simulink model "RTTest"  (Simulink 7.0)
settings: Solver=FixedStepDiscrete  StartTime=0.0  StopTime=inf  RelTol=1e-3
PreLoadFcn:
  | scramInitialize;
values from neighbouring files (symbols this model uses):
  nActSts = nAct    (= 5)    [scramInitialize.m]
  nAdcUSts = nAdcU    (= 18)    [scramInitialize.m]
  nDoutSts = nDout    (= 4)    [scramInitialize.m]
  nEncUSts = nEncU    (= 4)    [scramInitialize.m]
  nodeMats = node    [scramInitialize.m]
  nodeSts = node    [scramInitialize.m]
  nTblMats = nTbl    (= 6)    [scramInitialize.m]
  samplePeriod = 1/1024    (= 0.0009765625)    [scramInitialize.m]    (also in viewer.m = eval(getHeaderValue(header, 'DELTA_T')))
undefined symbols (not defined in the file or in its folder): DiscIntNeverNeededParam, Flat
libraries: xpcsystranlib x5, xpclib x5, simulink x1

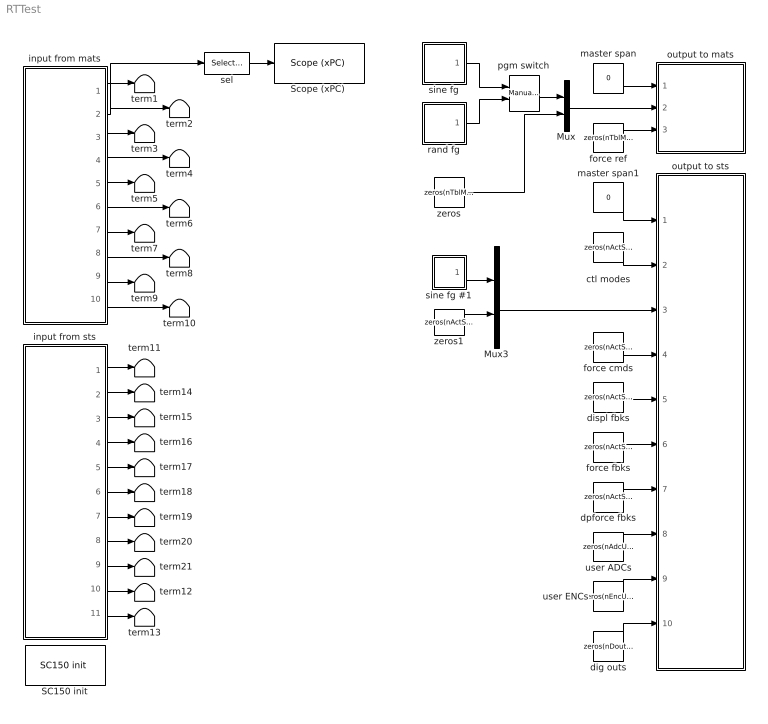
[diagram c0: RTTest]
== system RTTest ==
  Mux : Mux  Inputs=2
  Mux3 : Mux  Inputs=2
  SC150 init : xpcsystranlib/Shared Memory/SC150 init   node=node  pci=-1
  "Scope (xPC) " : xpclib/Misc./Scope (xPC)   SystemSampleTime=-1  scopeno=1  scopetype=Target  autostart=on  viewmode=Graphical redraw  formatstr='%15.6f'  grid=on  ylimits=[0,0]  nosamples=1024  noprepostsamples=0  interleave=1  triggermode=FreeRun  triggersignal=1  triggerlevel=0.0  triggerslope=Either  triggerscope=1  triggersample=0  filename=data.dat  mode=Lazy  writesize=512  autorestart=off
  ctl modes : Constant  Value=zeros(nActSts, 1)  OutDataType=sfix(16)  OutScaling=2^0
  dig outs : Constant  Value=zeros(nDoutSts, 1)  OutDataTypeMode=uint32  OutDataType=sfix(16)  OutScaling=2^0
  displ fbks : Constant  Value=zeros(nActSts, 1)  OutDataType=sfix(16)  OutScaling=2^0
  dpforce fbks : Constant  Value=zeros(nActSts, 1)  OutDataType=sfix(16)  OutScaling=2^0
  force cmds : Constant  Value=zeros(nActSts, 1)  OutDataType=sfix(16)  OutScaling=2^0
  force fbks : Constant  Value=zeros(nActSts, 1)  OutDataType=sfix(16)  OutScaling=2^0
  force ref : Constant  Value=zeros(nTblMats, 1)  OutDataType=sfix(16)  OutScaling=2^0
  input from mats : Subsystem
  input from sts : Subsystem
  master span : Constant  Value=0  OutDataType=sfix(16)  OutScaling=2^0
  master span1 : Constant  Value=0  OutDataType=sfix(16)  OutScaling=2^0
  output to mats : Subsystem
  output to sts : Subsystem
  pgm switch : simulink/Signal Routing/Manual Switch  SystemSampleTime=-1  sw=1  action=0  varsize=off
  rand fg : Subsystem  mask(Random Function Generator){shape=Flat, ampl=0.05, minFreq=0, maxFreq=10, spanInterval=1, samplePeriod=samplePeriod, showFRF=off}
      mask prompts: ampl "RMS amplitude"; minFreq "Minimum frequency (Hz)"; maxFreq "Maximum frequency (Hz)"; spanInterval "Span interval (sec)"; samplePeriod "Sample period (sec)"; showFRF "Show filter frequency response"
      mask init:
      | fsamp	= 1 / samplePeriod;
      | 
      | % design shaping filter
      | switch (shape)
      | 	case '1/F^2'	% 1/f^2 (two-pole lowpass)
      | 		% Note: Has unity amplitude at minFreq, then
      | 		% decreases at -40db per decade up to maxFreq.
      | 		minFreq = max(minFreq, 0.01*maxFreq);
      | 		k		= 0.1;
      | 		fpass	= k * minFreq;
      | 		alpha	= -exp(-2 * pi * fpass / fsamp);
      | 		a1		= 2 * alpha;
      | 		a2		= alpha^2;
      | 		b0		= (1/k)^2 * (1 + a1 + a2) * 0.25;
      | 		b1		= 2 * b0
      | 		b2		= b0
      | 		noiseBw = (minFreq / 3) * (1 - (minFreq / maxFreq)^3);
      | 	case '1/F'		% 1/f (one-pole lowpass)
      | 		% Note: Has unity amplitude at minFreq, then
      | 		% decreases at -20db per decade up to maxFreq.
      | 		minFreq = max(minFreq, 0.01*maxFreq);
      | 		k		= 0.1;
      | 		fpass	= k * minFreq;
      | 		alpha	= -exp(-2 * pi * fpass / fsamp);
      | 		a1		= alpha;
      | 		a2		= 0;
      | 		b0		= (1/k) * (1 + a1) * 0.5;
      | 		b1		= b0;
      | 		b2		= 0;
      | 		noiseBw = minFreq * (1 - (minFreq / maxFreq));
      | 	case 'Flat'		% flat
      | 		fpass	= maxFreq;
      | 		a1		= 0;
      | 		a2		= 0;
      | 		b0		= 1;
      | 		b1		= 0;
      | 		b2		= 0;
      | 		noiseBw = maxFreq - minFreq;
      | 	case 'F'		% f (single differentiator)
      | 		% Note:  A simple backward difference is a valid
      | 		% differentiator only up to about one half of nyquist.
      | 		% So we will select coefficients so that the slope,
      | 		% if extrapolated, would reach unity gain at nyquist
      | 		% (in reality, the gain will fall short of unity).
      | 		% These coefficients will be experimentally determined.
      | 		a1		= 0;
      | 		a2		= 0;
      | 		b0		= 0.33;
      | 		b1		= -b0;
      | 		b2		= 0;
      | 		noiseBw	= (4/3) * (maxFreq*(maxFreq/fsamp)^2 - minFreq*(minFreq/fsamp)^2);
      | 	case 'F^2'		% f^2 (double differentiator)
      | 		% Note:  See note above.
      | 		a1		= 0;
      | 		a2		= 0;
      | 		b0		= (0.33)^2;
      | 		b1		= -2 * b0;
      | 		b2		= b0;
      | 		noiseBw = (16/5) * (maxFreq*(maxFreq/fsamp)^4 - minFreq*(minFreq/fsamp)^4);
      | end
      | aSpf = [1 a1 a2];
      | bSpf = [b0 b1 b2];
      | peakAmpl = ampl * sqrt(3) * sqrt(max(0.5*fsamp/noiseBw, 1));
      | 
      | % design bandlimiting filter
      | fpassU	= maxFreq;
      | fstopU	= fpassU * 1.25;
      | fpassL	= min(minFreq, fpassU-0.001);
      | fstopL	= fpassL * 0.5;
      | rpass	= 0.01;
      | rstop	= 0.01;
      | rpassDB	= -20*log10(1-rpass);
      | rstopDB	= -20*log10(rstop);
      | bHpf	= [1];
      | aHpf	= [1];
      | bLpf	= [1];
      | aLpf	= [1];
      | if fpassL == 0
      | 		if fstopU < 0.5 * fsamp		% lowpass
      | 			[n, wn]	= ellipord(2*fpassU/fsamp, 2*fstopU/fsamp, rpassDB, rstopDB);
      | 			[bLpf, aLpf] = ellip(n, rpassDB, rstopDB, wn, 'low');
      | 		end
      | else
      | 		if fstopU < 0.5 * fsamp		% bandpass (implemented as series HP & LP)
      | 			rpassDB = rpassDB / 2;
      | 			[n, wn]	= ellipord(2*fpassU/fsamp, 2*fstopU/fsamp, rpassDB, rstopDB);
      | 			[bLpf, aLpf] = ellip(n, rpassDB, rstopDB, wn, 'low');
      | 			[n, wn]	= ellipord(2*fpassL/fsamp, 2*fstopL/fsamp, rpassDB, rstopDB);
      | 			[bHpf, aHpf] = ellip(n, rpassDB, rstopDB, wn, 'high');
      | 		else						% highpass
      | 			[n, wn]	= ellipord(2*fpassU/fsamp, 2*fstopU/fsamp, rpassDB, rstopDB);
      | 			[bHpf, aHpf] = ellip(n, rpassDB, rstopDB, wn, 'high');
      | 		end	
      | end
      | if showFRF
      | 	f     = linspace(0, fsamp/4, 8192);
      | 	tfSpf = freqz(bSpf, aSpf, f, fsamp);
      | 	tfLpf = freqz(bLpf, aLpf, f, fsamp);
      | 	tfHpf = freqz(bHpf, aHpf, f, fsamp);
      | 	plot(f, 20*log10(peakAmpl*abs(tfSpf.*tfLpf.*tfHpf)));
      | 	title('Filter Frequency Response');
      | 	ylabel('dB');
      | 	xlabel('Hz');
      | end
  sel : Selector  IndexOptions=Index vector (dialog)  Indices=1  OutputSizes=1
  sine fg : Subsystem  mask(Sine Function Generator){ampl=0.1, freq=5, spanInterval=1, samplePeriod=samplePeriod}
      mask prompts: ampl "Amplitude"; freq "Frequency (Hz)"; spanInterval "Span interval (sec)"; samplePeriod "Sample period (sec)"
  sine fg #1 : Subsystem  mask(Sine Function Generator){ampl=1, freq=1, spanInterval=1, samplePeriod=samplePeriod}
      mask prompts: ampl "Amplitude"; freq "Frequency (Hz)"; spanInterval "Span interval (sec)"; samplePeriod "Sample period (sec)"
  term{1..21} (21 alike) : Terminator
  user ADCs : Constant  Value=zeros(nAdcUSts, 1)  OutDataType=sfix(16)  OutScaling=2^0
  user ENCs : Constant  Value=zeros(nEncUSts, 1)  OutDataType=sfix(16)  OutScaling=2^0
  zeros : Constant  Value=zeros(nTblMats-1, 1)  OutDataType=sfix(16)  OutScaling=2^0
  zeros1 : Constant  Value=zeros(nActSts-1,1)  OutDataType=sfix(16)  OutScaling=2^0
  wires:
  master span/1 -> output to mats/1(master span)
  input from mats/1(master span) -> term1/1
  input from mats/2(displ ref) -> term2/1, sel/1
  input from mats/3(veloc ref) -> term3/1
  input from mats/4(force ref) -> term4/1
  sel/1 -> "Scope (xPC) "/1
  sine fg/1(out) -> pgm switch/1
  rand fg/1(out) -> pgm switch/2
  pgm switch/1 -> Mux/1
  zeros/1 -> Mux/2
  Mux/1 -> output to mats/2(displ ref)
  force ref/1 -> output to mats/3(force ref)
  input from mats/5(displ fbk) -> term5/1
  input from mats/6(veloc fbk) -> term6/1
  input from mats/7(force fbk) -> term7/1
  input from mats/8(comp fbk) -> term8/1
  input from mats/9(press fbk) -> term9/1
  input from mats/10(user adcs) -> term10/1
  input from sts/1(master span) -> term11/1
  input from sts/2(ctl modes) -> term14/1
  input from sts/3(displ cmds) -> term15/1
  input from sts/4(force cmds) -> term16/1
  input from sts/5(displ fbks) -> term17/1
  input from sts/6(force fbks) -> term18/1
  input from sts/7(dpforce fbks) -> term19/1
  input from sts/8(valve cmds) -> term20/1
  input from sts/9(user adcs) -> term21/1
  input from sts/10(user encs) -> term12/1
  input from sts/11(dig inps) -> term13/1
  master span1/1 -> output to sts/1(master span)
  ctl modes/1 -> output to sts/2(ctl modes)
  force cmds/1 -> output to sts/4(force cmds)
  Mux3/1 -> output to sts/3(displ cmds)
  displ fbks/1 -> output to sts/5(displ fbks)
  force fbks/1 -> output to sts/6(force fbks)
  dpforce fbks/1 -> output to sts/7(dpforce fbks)
  user ADCs/1 -> output to sts/8(user adcs)
  dig outs/1 -> output to sts/10(dig outs)
  user ENCs/1 -> output to sts/9(user encs)
  sine fg #1/1(out) -> Mux3/1
  zeros1/1 -> Mux3/2

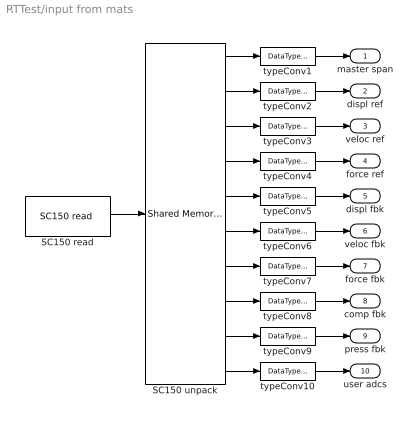
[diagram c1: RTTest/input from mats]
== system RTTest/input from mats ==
  SC150 read : xpcsystranlib/Shared Memory/SC150 read   partition=nodeMats.Partitions(4:end)  errorport=off  ts=samplePeriod  pci=-1
  SC150 unpack : xpclib/Shared Memory/Shared Memory Unpack   partition=nodeMats.Partitions(4:end)
  typeConv{1..10} (10 alike) : DataTypeConversion  OutDataTypeMode=double  OutDataType=sfix(16)  OutScaling=2^0
  master span : Outport  OutDataType=sfix(16)  OutScaling=2^0
  displ ref : Outport  Port=2  OutDataType=sfix(16)  OutScaling=2^0
  veloc ref : Outport  Port=3  OutDataType=sfix(16)  OutScaling=2^0
  force ref : Outport  Port=4  OutDataType=sfix(16)  OutScaling=2^0
  displ fbk : Outport  Port=5  OutDataType=sfix(16)  OutScaling=2^0
  veloc fbk : Outport  Port=6  OutDataType=sfix(16)  OutScaling=2^0
  force fbk : Outport  Port=7  OutDataType=sfix(16)  OutScaling=2^0
  comp fbk : Outport  Port=8  OutDataType=sfix(16)  OutScaling=2^0
  press fbk : Outport  Port=9  OutDataType=sfix(16)  OutScaling=2^0
  user adcs : Outport  Port=10  OutDataType=sfix(16)  OutScaling=2^0
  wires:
  SC150 read/1 -> SC150 unpack/1
  typeConv1/1 -> master span/1
  typeConv2/1 -> displ ref/1
  typeConv3/1 -> veloc ref/1
  typeConv4/1 -> force ref/1
  SC150 unpack/1 -> typeConv1/1
  SC150 unpack/2 -> typeConv2/1
  SC150 unpack/3 -> typeConv3/1
  SC150 unpack/4 -> typeConv4/1
  SC150 unpack/5 -> typeConv5/1
  SC150 unpack/6 -> typeConv6/1
  typeConv5/1 -> displ fbk/1
  typeConv6/1 -> veloc fbk/1
  SC150 unpack/7 -> typeConv7/1
  SC150 unpack/8 -> typeConv8/1
  SC150 unpack/9 -> typeConv9/1
  SC150 unpack/10 -> typeConv10/1
  typeConv10/1 -> user adcs/1
  typeConv9/1 -> press fbk/1
  typeConv8/1 -> comp fbk/1
  typeConv7/1 -> force fbk/1

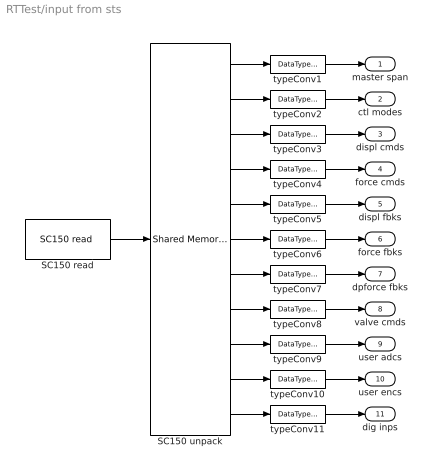
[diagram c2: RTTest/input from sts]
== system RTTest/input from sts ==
  SC150 read : xpcsystranlib/Shared Memory/SC150 read   partition=nodeSts.Partitions(11:21)  errorport=off  ts=samplePeriod  pci=-1
  SC150 unpack : xpclib/Shared Memory/Shared Memory Unpack   partition=nodeSts.Partitions(11:21)
  typeConv{1,3..10} (9 alike) : DataTypeConversion  OutDataTypeMode=double  OutDataType=sfix(16)  OutScaling=2^0
  typeConv11 : DataTypeConversion  OutDataTypeMode=uint32  OutDataType=sfix(16)  OutScaling=2^0
  typeConv2 : DataTypeConversion  OutDataTypeMode=uint32  OutDataType=sfix(16)  OutScaling=2^0
  master span : Outport  OutDataType=sfix(16)  OutScaling=2^0
  ctl modes : Outport  Port=2  OutDataType=sfix(16)  OutScaling=2^0
  displ cmds : Outport  Port=3  OutDataType=sfix(16)  OutScaling=2^0
  force cmds : Outport  Port=4  OutDataType=sfix(16)  OutScaling=2^0
  displ fbks : Outport  Port=5  OutDataType=sfix(16)  OutScaling=2^0
  force fbks : Outport  Port=6  OutDataType=sfix(16)  OutScaling=2^0
  dpforce fbks : Outport  Port=7  OutDataType=sfix(16)  OutScaling=2^0
  valve cmds : Outport  Port=8  OutDataType=sfix(16)  OutScaling=2^0
  user adcs : Outport  Port=9  OutDataType=sfix(16)  OutScaling=2^0
  user encs : Outport  Port=10  OutDataType=sfix(16)  OutScaling=2^0
  dig inps : Outport  Port=11  OutDataType=sfix(16)  OutScaling=2^0
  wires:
  typeConv10/1 -> user encs/1
  SC150 unpack/10 -> typeConv10/1
  SC150 unpack/11 -> typeConv11/1
  typeConv11/1 -> dig inps/1
  typeConv9/1 -> user adcs/1
  typeConv8/1 -> valve cmds/1
  typeConv7/1 -> dpforce fbks/1
  typeConv6/1 -> force fbks/1
  typeConv5/1 -> displ fbks/1
  typeConv4/1 -> force cmds/1
  typeConv3/1 -> displ cmds/1
  typeConv1/1 -> master span/1
  SC150 read/1 -> SC150 unpack/1
  typeConv2/1 -> ctl modes/1
  SC150 unpack/1 -> typeConv1/1
  SC150 unpack/2 -> typeConv2/1
  SC150 unpack/3 -> typeConv3/1
  SC150 unpack/4 -> typeConv4/1
  SC150 unpack/5 -> typeConv5/1
  SC150 unpack/6 -> typeConv6/1
  SC150 unpack/7 -> typeConv7/1
  SC150 unpack/8 -> typeConv8/1
  SC150 unpack/9 -> typeConv9/1

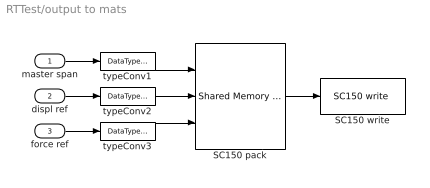
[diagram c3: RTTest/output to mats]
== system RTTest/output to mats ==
  master span : Inport  OutDataType=sfix(16)  OutScaling=2^0
  displ ref : Inport  Port=2  OutDataType=sfix(16)  OutScaling=2^0
  force ref : Inport  Port=3  OutDataType=sfix(16)  OutScaling=2^0
  SC150 pack : xpclib/Shared Memory/Shared Memory Pack   partition=nodeMats.Partitions(1:3)
  SC150 write : xpcsystranlib/Shared Memory/SC150 write   partition=nodeMats.Partitions(1:3)  errorport=off  ts=samplePeriod  pci=-1
  typeConv1 : DataTypeConversion  OutDataTypeMode=single  OutDataType=sfix(16)  OutScaling=2^0
  typeConv2 : DataTypeConversion  OutDataTypeMode=single  OutDataType=sfix(16)  OutScaling=2^0
  typeConv3 : DataTypeConversion  OutDataTypeMode=single  OutDataType=sfix(16)  OutScaling=2^0
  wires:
  master span/1 -> typeConv1/1
  displ ref/1 -> typeConv2/1
  SC150 pack/1 -> SC150 write/1
  typeConv1/1 -> SC150 pack/1
  typeConv2/1 -> SC150 pack/2
  force ref/1 -> typeConv3/1
  typeConv3/1 -> SC150 pack/3

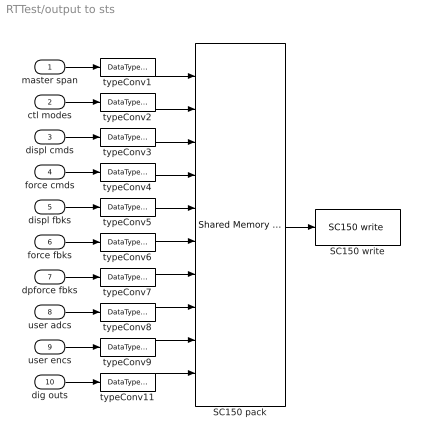
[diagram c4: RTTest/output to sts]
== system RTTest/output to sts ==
  master span : Inport  OutDataType=sfix(16)  OutScaling=2^0
  ctl modes : Inport  Port=2  OutDataType=sfix(16)  OutScaling=2^0
  displ cmds : Inport  Port=3  OutDataType=sfix(16)  OutScaling=2^0
  force cmds : Inport  Port=4  OutDataType=sfix(16)  OutScaling=2^0
  displ fbks : Inport  Port=5  OutDataType=sfix(16)  OutScaling=2^0
  force fbks : Inport  Port=6  OutDataType=sfix(16)  OutScaling=2^0
  dpforce fbks : Inport  Port=7  OutDataType=sfix(16)  OutScaling=2^0
  user adcs : Inport  Port=8  OutDataType=sfix(16)  OutScaling=2^0
  user encs : Inport  Port=9  OutDataType=sfix(16)  OutScaling=2^0
  dig outs : Inport  Port=10  OutDataType=sfix(16)  OutScaling=2^0
  SC150 pack : xpclib/Shared Memory/Shared Memory Pack   partition=nodeSts.Partitions(1:10)
  SC150 write : xpcsystranlib/Shared Memory/SC150 write   partition=nodeSts.Partitions(1:10)  errorport=off  ts=samplePeriod  pci=-1
  typeConv{1,3..9} (8 alike) : DataTypeConversion  OutDataTypeMode=single  OutDataType=sfix(16)  OutScaling=2^0
  typeConv11 : DataTypeConversion  OutDataTypeMode=uint32  OutDataType=sfix(16)  OutScaling=2^0
  typeConv2 : DataTypeConversion  OutDataTypeMode=uint32  OutDataType=sfix(16)  OutScaling=2^0
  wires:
  typeConv9/1 -> SC150 pack/9
  user encs/1 -> typeConv9/1
  typeConv11/1 -> SC150 pack/10
  typeConv8/1 -> SC150 pack/8
  typeConv7/1 -> SC150 pack/7
  typeConv6/1 -> SC150 pack/6
  typeConv5/1 -> SC150 pack/5
  dig outs/1 -> typeConv11/1
  user adcs/1 -> typeConv8/1
  dpforce fbks/1 -> typeConv7/1
  force fbks/1 -> typeConv6/1
  displ fbks/1 -> typeConv5/1
  force cmds/1 -> typeConv4/1
  master span/1 -> typeConv1/1
  SC150 pack/1 -> SC150 write/1
  displ cmds/1 -> typeConv3/1
  ctl modes/1 -> typeConv2/1
  typeConv1/1 -> SC150 pack/1
  typeConv2/1 -> SC150 pack/2
  typeConv3/1 -> SC150 pack/3
  typeConv4/1 -> SC150 pack/4

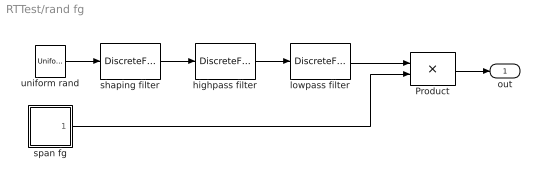
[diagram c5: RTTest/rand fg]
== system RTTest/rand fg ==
  Product : Product  OutDataType=sfix(16)  OutScaling=2^0
  highpass filter : DiscreteFilter  Numerator=bHpf  Denominator=aHpf  SampleTime=samplePeriod
  lowpass filter : DiscreteFilter  Numerator=bLpf  Denominator=aLpf  SampleTime=samplePeriod
  shaping filter : DiscreteFilter  Numerator=bSpf  Denominator=aSpf  SampleTime=samplePeriod
  span fg : Subsystem  mask{spanInterval=spanInterval, samplePeriod=samplePeriod}
      mask prompts: spanInterval "Span interval (sec)"; samplePeriod "Sample period (sec)"
  uniform rand : UniformRandomNumber  Minimum=-peakAmpl  Maximum=peakAmpl  SampleTime=samplePeriod
  out : Outport  OutDataType=sfix(16)  OutScaling=2^0
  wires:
  lowpass filter/1 -> Product/1
  highpass filter/1 -> lowpass filter/1
  shaping filter/1 -> highpass filter/1
  uniform rand/1 -> shaping filter/1
  Product/1 -> out/1
  span fg/1(out) -> Product/2

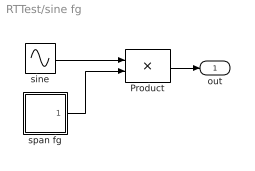
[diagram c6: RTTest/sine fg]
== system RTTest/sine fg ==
  Product : Product  OutDataType=sfix(16)  OutScaling=2^0
  sine : Sin  Amplitude=ampl  Frequency=2 * pi * freq  SampleTime=samplePeriod
  span fg : Subsystem  mask{spanInterval=spanInterval, samplePeriod=samplePeriod}
      mask prompts: spanInterval "Span interval (sec)"; samplePeriod "Sample period (sec)"
  out : Outport  OutDataType=sfix(16)  OutScaling=2^0
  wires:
  span fg/1(out) -> Product/2
  sine/1 -> Product/1
  Product/1 -> out/1

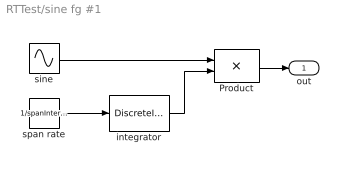
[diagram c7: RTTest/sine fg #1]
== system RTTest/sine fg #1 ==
  Product : Product  OutDataType=sfix(16)  OutScaling=2^0
  integrator : DiscreteIntegrator  SampleTime=-1  OutDataType=sfix(16)  OutScaling=2^0  LimitOutput=on  UpperSaturationLimit=1  LowerSaturationLimit=0  ICPrevOutput=DiscIntNeverNeededParam  ICPrevScaledInput=DiscIntNeverNeededParam
  sine : Sin  Amplitude=ampl  Frequency=2 * pi * freq  SampleTime=samplePeriod
  span rate : Constant  Value=1/spanInterval  OutDataType=sfix(16)  OutScaling=2^0
  out : Outport  OutDataType=sfix(16)  OutScaling=2^0
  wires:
  Product/1 -> out/1
  sine/1 -> Product/1
  span rate/1 -> integrator/1
  integrator/1 -> Product/2

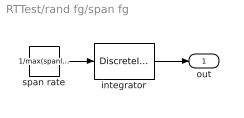
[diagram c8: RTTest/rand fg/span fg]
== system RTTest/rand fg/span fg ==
  integrator : DiscreteIntegrator  SampleTime=samplePeriod  OutDataType=sfix(16)  OutScaling=2^0  LimitOutput=on  UpperSaturationLimit=1  LowerSaturationLimit=0  ICPrevOutput=DiscIntNeverNeededParam  ICPrevScaledInput=DiscIntNeverNeededParam
  span rate : Constant  Value=1/max(spanInterval,samplePeriod)  OutDataType=sfix(16)  OutScaling=2^0  SampleTime=samplePeriod
  out : Outport  OutDataType=sfix(16)  OutScaling=2^0
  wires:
  integrator/1 -> out/1
  span rate/1 -> integrator/1

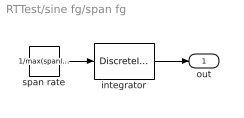
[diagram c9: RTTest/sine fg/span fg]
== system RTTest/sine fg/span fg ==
  integrator : DiscreteIntegrator  SampleTime=samplePeriod  OutDataType=sfix(16)  OutScaling=2^0  LimitOutput=on  UpperSaturationLimit=1  LowerSaturationLimit=0  ICPrevOutput=DiscIntNeverNeededParam  ICPrevScaledInput=DiscIntNeverNeededParam
  span rate : Constant  Value=1/max(spanInterval,samplePeriod)  OutDataType=sfix(16)  OutScaling=2^0  SampleTime=samplePeriod
  out : Outport  OutDataType=sfix(16)  OutScaling=2^0
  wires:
  integrator/1 -> out/1
  span rate/1 -> integrator/1
